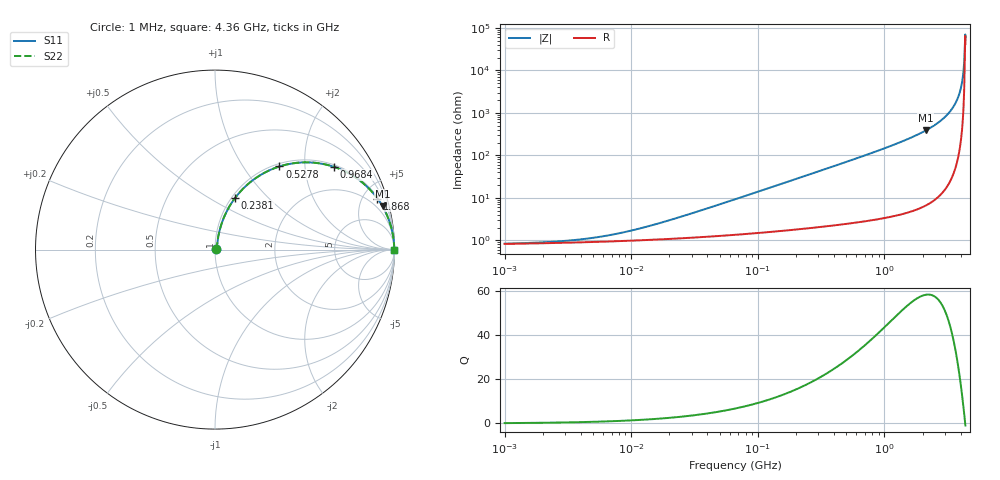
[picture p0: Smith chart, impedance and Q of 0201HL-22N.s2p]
# MHz  S  MA  R  50
!Freq  MagS11  AngS11  MagS21  AngS21  MagS12  AngS12  MagS22  AngS22
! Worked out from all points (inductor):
!   844 points, 1 MHz to 4.36 GHz, reference 50 ohm
!   read as one part in series: L = 22 nH near 24.15 MHz
!   highest Q = 58.4 at 2.125 GHz (marker M1), where L = 28.9 nH
!   self-resonance near 4.308 GHz
!   S11 on the Smith chart (normalised r, x): 1 MHz: 1.02, +0.00; 238.1 MHz: 1.04, +0.66; 527.8 MHz: 1.05, +1.48; 968.4 MHz: 1.07, +2.82; 1.868 GHz: 1.11, +6.33; 4.36 GHz: open
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1  0.008282 9.4  0.9918 -0.1  0.9918 -0.1  0.008282 9.4
4.06737  0.0105 31.7  0.9911 -0.3  0.9911 -0.3  0.0105 31.7
7.922199  0.0144 48.2  0.9905 -0.6  0.9905 -0.6  0.0144 48.2
16.3797  0.02468 63.9  0.9894 -1.3  0.9894 -1.3  0.02468 63.9
66.62232  0.09148 76.5  0.9826 -5.2  0.9826 -5.2  0.09148 76.5
128.4785  0.173 75.0  0.9697 -9.9  0.9697 -9.9  0.173 75.0
238.0979  0.3087 68.8  0.9337 -18.0  0.9337 -18.0  0.3087 68.8
268.2947  0.3434 66.9  0.9213 -20.1  0.9213 -20.1  0.3434 66.9
527.7953  0.586 52.2  0.7909 -35.8  0.7909 -35.8  0.586 52.2
968.4323  0.8067 34.9  0.5725 -53.8  0.5725 -53.8  0.8067 34.9
1080.449  0.8386 31.8  0.5267 -57.0  0.5267 -57.0  0.8386 31.8
1867.583  0.9488 17.4  0.2996 -71.6  0.2996 -71.6  0.9488 17.4
2125.484  0.9641 14.5  0.2496 -74.6  0.2496 -74.6  0.9641 14.5
3010.966  0.9899 7.1  0.1236 -81.8  0.1236 -81.8  0.9899 7.1
3392.832  0.9946 4.7  0.08274 -83.9  0.08274 -83.9  0.9946 4.7
3710.691  0.9969 3.0  0.05259 -85.1  0.05259 -85.1  0.9969 3.0
3899.973  0.9978 2.1  0.03596 -85.4  0.03596 -85.4  0.9978 2.1
4058.328  0.9983 1.3  0.02271 -84.9  0.02271 -84.9  0.9983 1.3
4139.9  0.9984 0.9  0.0161 -83.9  0.0161 -83.9  0.9984 0.9
4223.112  0.9986 0.5  0.00952 -81.0  0.00952 -81.0  0.9986 0.5
4351.077  0.9987 -0.0  0.001434 20.8  0.001434 20.8  0.9987 -0.0
4360  0.9987 -0.1  0.001791 41.7  0.001791 41.7  0.9987 -0.1
